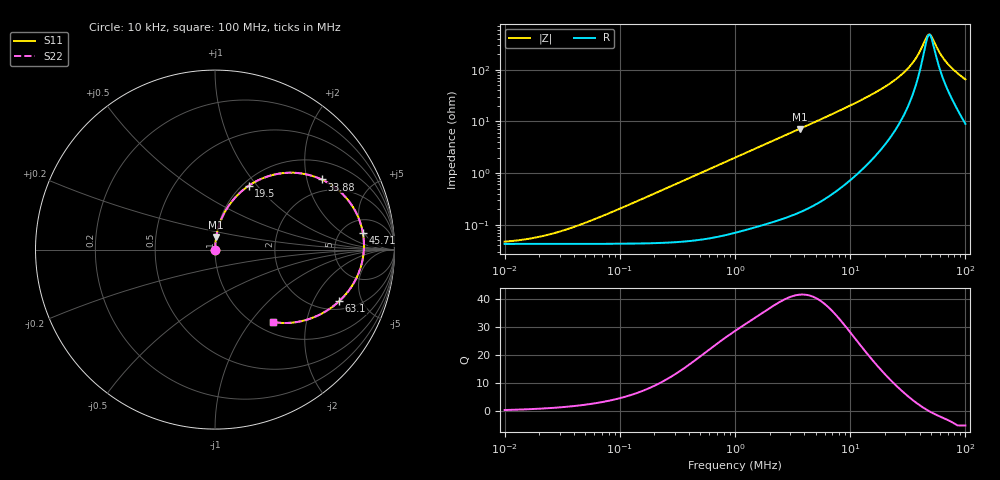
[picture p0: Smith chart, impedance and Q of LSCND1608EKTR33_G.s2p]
! LSCND1608EKTR33_G  S-PARAMETER MODEL  ( Standard Model )
! Model Generated by TAIYO YUDEN Corporation (http://www.ty-top.com)
! Version 1.0
! TAIYO YUDEN Control No. 231226
! Copyright(c) 2023 TAIYO YUDEN CO.,LTD. All Rights Reserved.
! Product Description (link to TY-COMPAS)
! https://ds.yuden.co.jp/TYCOMPAS/or/detail?pn=LSCND1608EKTR33MG&u=M
! Products Name : Inductors
! Characteristics :
!  Inductance : 0.33 [uH] , SRF(min) : - [Hz] , DC Resistance(max) : 47 [mOhm]
!  Rated Current : Saturation  3.0 [A] (dL = 30 [%]), Temp Rise  2.9 [A] (dT = 40 [degC])
!  Case Size : 1.6 x 0.8 / 0.063 x 0.031 [mm/inch] , Thickness : 0.5 / 0.02 [mm/inch]
!  (Conditions: Temperature = 25 [degC] , DC Bias Current = 0 [A])
! External Node Assignments :
!  1  o---GGG---o  2
! GND o---------o GND
! Frequency Range : 10kHz  -  100MHz  [ 402 STEP ]
# MHz S RI R 50
! Freq[MHz].  S11 Real  S11 Imag  S21 Real  S21 Imag  S12 Real  S12 Imag  S22 Real  S22 Imag
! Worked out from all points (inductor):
!   401 points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, 10 kHz to 100 MHz, reference 50 ohm
!   read as one part in series: L = 317 nH near 64.56 kHz
!   highest Q = 41.4 at 3.631 MHz (marker M1), where L = 313 nH
!   self-resonance near 48.77 MHz
!   S11 on the Smith chart (normalised r, x): 10 kHz: 1.00, +0.00; 19.5 MHz: 1.07, +0.90; 33.88 MHz: 1.56, +2.46; 45.71 MHz: 7.99, +4.65; 63.1 MHz: 2.47, -3.24; 100 MHz: 1.18, -1.29
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0.01  0.000423 0.000199  0.9996 -0.000199  0.9996 -0.000199  0.000423 0.000199
0.02138  0.000423 0.000426  0.9996 -0.000426  0.9996 -0.000426  0.000423 0.000426
0.046774  0.000424 0.000932  0.9996 -0.000932  0.9996 -0.000932  0.000424 0.000932
0.218776  0.00046 0.00435  0.9995 -0.00435  0.9995 -0.00435  0.00046 0.00435
1  0.00108 0.0198  0.9989 -0.0198  0.9989 -0.0198  0.00108 0.0198
3.630781  0.00676 0.0707  0.9932 -0.0707  0.9932 -0.0707  0.00676 0.0707
4.677351  0.0106 0.091  0.9894 -0.091  0.9894 -0.091  0.0106 0.091
11.48154  0.0611 0.2203  0.9389 -0.2203  0.9389 -0.2203  0.0611 0.2203
15.48817  0.1141 0.2919  0.8859 -0.2919  0.8859 -0.2919  0.1141 0.2919
19.49845  0.1873 0.3553  0.8127 -0.3553  0.8127 -0.3553  0.1873 0.3553
21.87762  0.2408 0.3864  0.7592 -0.3864  0.7592 -0.3864  0.2408 0.3864
28.18383  0.4159 0.4283  0.5841 -0.4283  0.5841 -0.4283  0.4159 0.4283
33.88442  0.5945 0.3907  0.4055 -0.3907  0.4055 -0.3907  0.5945 0.3907
38.90451  0.7299 0.2895  0.2701 -0.2895  0.2701 -0.2895  0.7299 0.2895
45.70882  0.8244 0.0908  0.1756 -0.0908  0.1756 -0.0908  0.8244 0.0908
47.86301  0.8301 0.0261  0.1699 -0.0261  0.1699 -0.0261  0.8301 0.0261
50.11872  0.8257 -0.0378  0.1743 0.0378  0.1743 0.0378  0.8257 -0.0378
56.23413  0.7762 -0.1812  0.2238 0.1812  0.2238 0.1812  0.7762 -0.1812
63.09573  0.6918 -0.2876  0.3082 0.2876  0.3082 0.2876  0.6918 -0.2876
69.1831  0.6145 -0.3454  0.3855 0.3454  0.3855 0.3454  0.6145 -0.3454
77.62471  0.5162 -0.3894  0.4838 0.3894  0.4838 0.3894  0.5162 -0.3894
100  0.3218 -0.4028  0.6782 0.4028  0.6782 0.4028  0.3218 -0.4028
